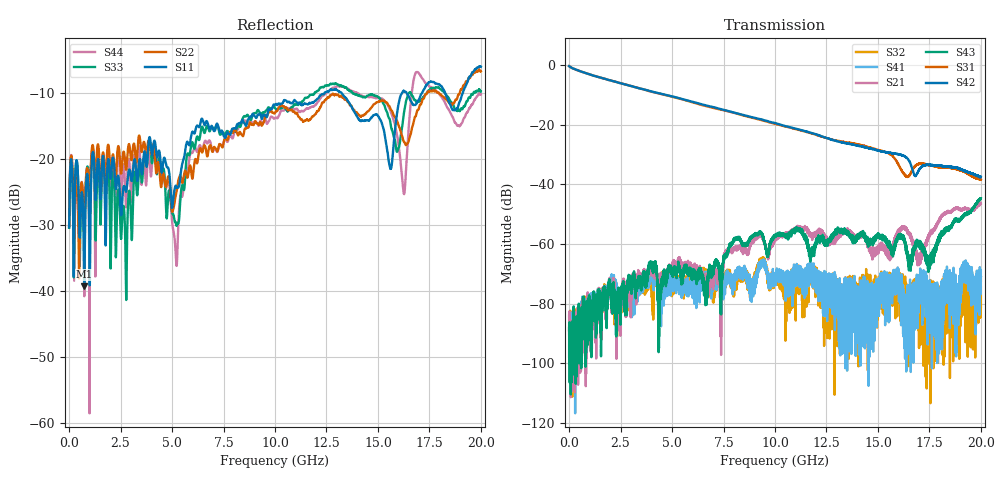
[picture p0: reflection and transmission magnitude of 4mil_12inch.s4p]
!Agilent Technologies,N5230A,US43500443,A.06.04.32
!Agilent N5230A: A.06.04.32
!Date: Wednesday, December 12, 2012 16:48:37
!Correction: S11(Full 4 Port(1,2,3,4)) S12(Full 4 Port(1,2,3,4)) S13(Full 4 Port(1,2,3,4)) S14(Full 4 Port(1,2,3,4)) S21(Full 4 Port(1,2,3,4)) S22(Full 4 Port(1,2,3,4)) S23(Full 4 Port(1,2,3,4)) S24(Full 4 Port(1,2,3,4)) S31(Full 4 Port(1,2,3,4)) S32(Full 4 Port(1,2,3,4)) S33(Full 4 Port(1,2,3,4)) S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
!S4P File: Measurements: <S11,S12,S13,S14>, <S21,S22,S23,S24>, <S31,S32,S33,S34>, <S41,S42,S43,S44>:
# Hz S  dB  R 50
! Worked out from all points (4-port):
!   10000 points, 1 MHz to 20 GHz, reference 50 ohm
!   strongest paths, dB at 1 MHz, 5.001 GHz, 10 GHz, 15 GHz, 20 GHz:
!     S42: -0.3, -10.4, -19.4, -28.6, -37.5
!     S31: -0.3, -10.5, -19.6, -28.4, -38.3
!     S43: -89.0, -70.0, -57.0, -56.6, -44.6
!     S21: -84.0, -67.2, -58.2, -60.8, -46.4
!     S41: -97.8, -73.4, -70.4, -78.4, -71.0
!     S32: -88.0, -73.4, -72.7, -80.8, -81.1
!   lowest |S11| = -39.3 dB at 735 MHz (marker M1), VSWR 1.02, Z = 49.2 - j0.707 ohm
!   |S11| at or under -10 dB: start of sweep to 12.4 GHz; 13.24 GHz to 16.17 GHz (2.932 GHz wide, 19.9 % of centre); 18.26 GHz to 19.12 GHz (854.4 MHz wide, 4.57 % of centre)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
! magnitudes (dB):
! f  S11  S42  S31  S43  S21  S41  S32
! 1 MHz  -30.4  -0.3  -0.3  -89.0  -84.0  -97.8  -88.0
! 735 MHz  -39.3  -2.4  -2.4  -84.5  -81.3  -82.0  -81.1
! 7.345 GHz  -15.9  -14.7  -14.8  -72.8  -76.1  -71.1  -69.2
! 9.261 GHz  -13.1  -18.1  -18.3  -55.9  -57.0  -66.0  -65.7
! 16.26 GHz  -9.7  -30.4  -36.4  -58.2  -54.7  -84.5  -82.3
! 17.48 GHz  -8.3  -33.5  -33.5  -65.7  -57.7  -81.2  -83.6
! 20 GHz  -6.0  -37.5  -38.3  -44.6  -46.4  -71.0  -81.1
